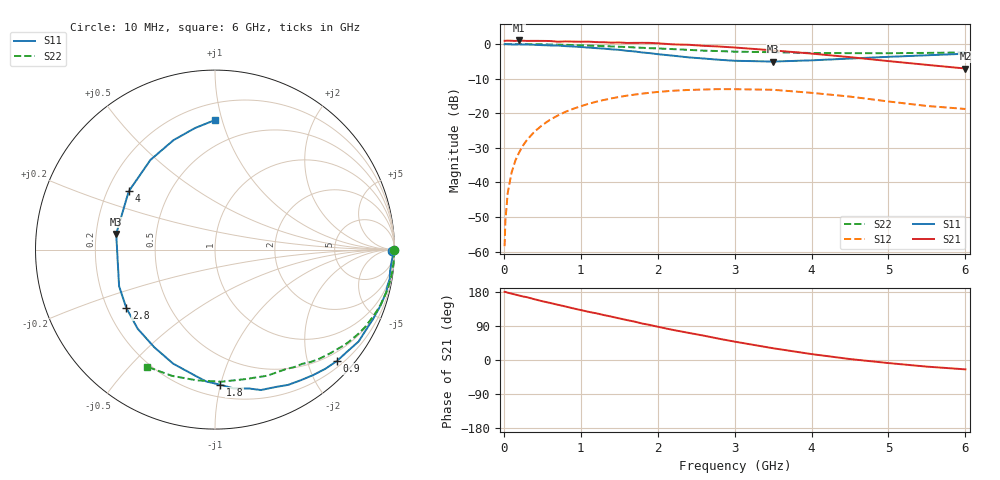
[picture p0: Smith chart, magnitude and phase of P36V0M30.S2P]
! SIEMENS Small Signal Semiconductors
! BFP181
! Si NPN RF Bipolar Junction Transistor in SOT143
! VCE = 6 V  IC = 0.3 mA
! Common Emitter S-Parameters:  March  1996
# GHz  S  MA  R  50
!  f  S11  S21  S12  S22
! GHz  MAG  ANG  MAG  ANG  MAG  ANG  MAG  ANG
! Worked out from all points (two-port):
!   36 points, 10 MHz to 6 GHz, reference 50 ohm
!   highest |S21| = 1.02 dB at 200 MHz (marker M1); lowest = -7.1 dB at 6 GHz (marker M2)
!   |S21| within 3 dB of the highest: start of sweep to 3.571 GHz
!   lowest |S11| = -5.1 dB at 3.5 GHz (marker M3), VSWR 3.52, Z = 14.3 + j3.62 ohm
!   |S11| at or under -10 dB: nowhere
!   |S22| runs from -2.7 to 0.0 dB; largest |S21 - S12| = 1.1
!   S11 on the Smith chart (normalised r, x): 10 MHz: open; 900 MHz: 0.31, -2.54; 1.8 GHz: 0.29, -1.00; 2.8 GHz: 0.28, -0.28; 4 GHz: 0.29, +0.28; 6 GHz: 0.31, +0.95
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0.01  0.988 -0.6  1.111 179.8  0.0012 86.3  0.9989 -0.2
0.02  0.9939 -0.9  1.111 179.7  0.0028 85.2  0.9978 -0.4
0.05  0.9901 -2.3  1.118 177.7  0.007 89.3  0.998 -1.2
0.1  0.9848 -4.7  1.112 175.1  0.0138 86.3  0.9979 -2.4
0.15  0.9827 -7.1  1.106 172.7  0.0207 84.1  0.9977 -3.5
0.2  0.9873 -9.5  1.124 170.1  0.0273 83.3  0.9972 -4.6
0.3  0.983 -13.9  1.107 165.8  0.041 79.5  0.9952 -7.0
0.5  0.9619 -23.7  1.107 155.1  0.0672 72.4  0.9887 -11.8
0.9  0.92 -42.4  1.083 136.3  0.1156 58.5  0.9646 -20.7
1.1  0.887 -52.1  1.081 127.2  0.1366 52.1  0.9481 -25.0
1.5  0.8231 -71.9  1.052 109.8  0.1718 39.4  0.9117 -33.2
1.8  0.753 -87.9  1.039 96.2  0.1918 30.9  0.8806 -38.8
2  0.7125 -98.6  1.023 87.8  0.2028 25.2  0.8619 -42.3
2.2  0.677 -110.1  0.986 79.3  0.2111 19.5  0.8422 -46.1
2.4  0.6407 -121.9  0.974 71.7  0.2167 14.0  0.8223 -49.6
2.8  0.5912 -146.8  0.919 56.0  0.2228 4.1  0.7897 -56.0
3  0.5719 -159.1  0.889 48.5  0.2221 -0.9  0.7741 -59.3
3.5  0.5572 171.0  0.808 31.0  0.2179 -11.9  0.7605 -67.5
4  0.58 146.0  0.726 15.6  0.1969 -21.0  0.7408 -77.0
4.5  0.6155 125.8  0.645 2.5  0.1737 -28.0  0.737 -87.3
5.5  0.6865 99.3  0.499 -17.5  0.1272 -29.5  0.7431 -108.8
6  0.7228 89.8  0.442 -24.7  0.1151 -24.4  0.7543 -120.0
